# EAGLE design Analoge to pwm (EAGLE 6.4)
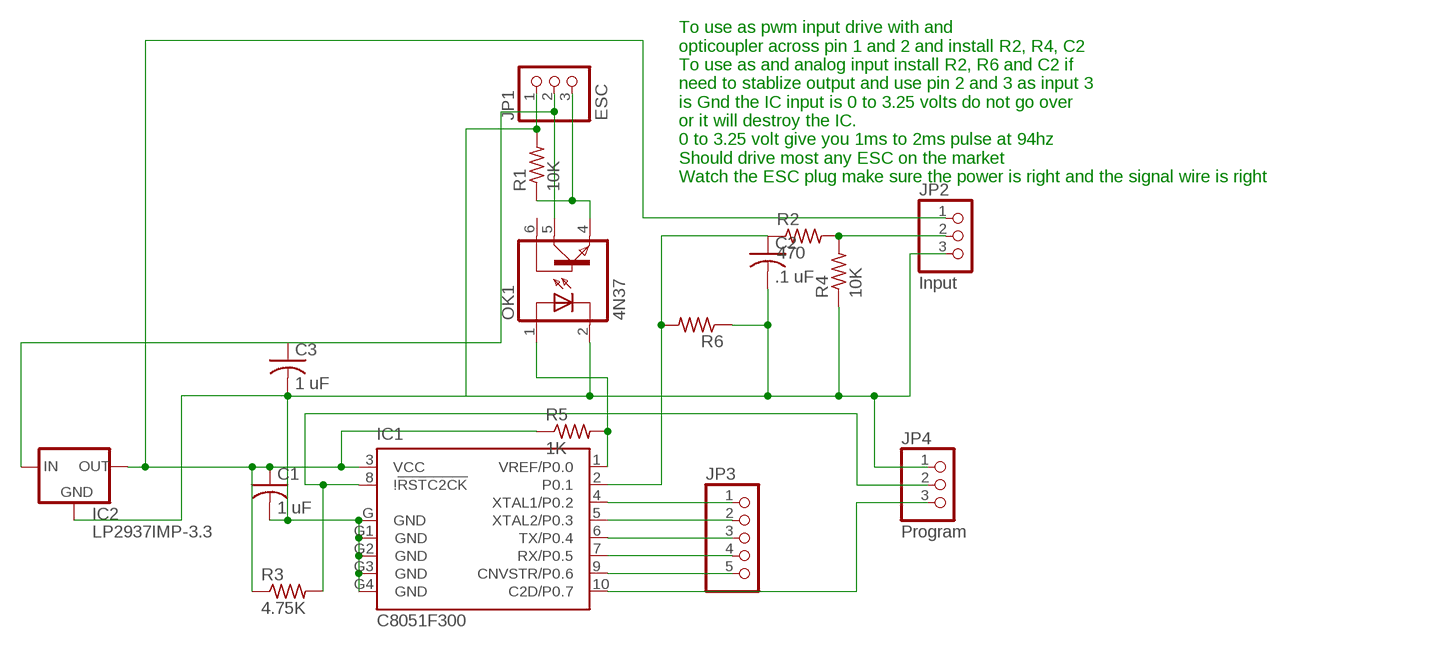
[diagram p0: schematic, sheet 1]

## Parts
C1  1 uF  C-USC0805  [C0805]
C2  .1 uF  C-USC0805  [C0805]
C3  1 uF  C-USC0805  [C0805]
IC1  C8051F300  [MLP11]
IC2  LP2937IMP-3.3  LP2950CDT-3.3  [DPACK]
JP1  ESC  PINHD-1X3  [1X03]
JP2  Input  PINHD-1X3  [1X03]
JP3  PINHD-1X5  [1X05]
JP4  Program  PINHD-1X3  [1X03]
OK1  4N37  [DIL06]
R1  10K  R-US_R0805  [R0805]
R2  470  R-US_R0805  [R0805]
R3  4.75K  R-US_M0805  [M0805]
R4  10K  R-US_R0805  [R0805]
R5  1K  R-US_R0805  [R0805]
R6  R-US_R0805  [R0805]

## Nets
N$1: IC1.10(C2D/P0.7) JP4.3
N$2: IC1.8(!!RSTC2CK) JP4.2 R3.2
N$4: IC1.1(VREF/P0.0) OK1.1(A) R5.2
N$6: C3.1 IC2.1(IN) JP1.2 OK1.5(COL)
N$7: JP1.3 OK1.4(EMI) R1.1
N$8: C1.2 C2.2 C3.2 IC1.G1(GND) IC1.G2(GND) IC1.G3(GND) IC1.G4(GND) IC1.G(GND) IC2.4(GND) JP1.1 JP2.3 JP4.1 OK1.2(C) R1.2 R4.1 R6.1
N$9: C2.1 IC1.2(P0.1) R2.1 R6.2
N$10: JP2.2 R2.2 R4.2
N$12: IC1.4(XTAL1/P0.2) JP3.1
N$13: IC1.5(XTAL2/P0.3) JP3.2
N$14: IC1.6(TX/P0.4) JP3.3
N$15: IC1.7(RX/P0.5) JP3.4
N$16: IC1.9(CNVSTR/P0.6) JP3.5
N$17: C1.1 IC1.3(VCC) IC2.3(OUT) JP2.1 R3.1 R5.1
Unconnected: OK1.6(BAS)

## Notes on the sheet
- To use as pwm input drive with and 
  opticoupler across pin 1 and 2 and install R2, R4, C2  
  To use as and analog input install R2, R6 and C2 if
  need to stablize output and use pin 2 and 3 as input 3 
  is Gnd the IC input is 0 to 3.25 volts do not go over
  or it will destroy the IC.
  0 to 3.25 volt give you 1ms to 2ms pulse at 94hz
  Should drive most any ESC on the market
  Watch the ESC plug make sure the power is right and the signal wire is right

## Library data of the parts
C1-C3 = resistor:C-US: CAPACITOR, American symbol
IC1 = silabs:C8051F30*: 25 MIPS, 8 kB Flash, 8-Bit ADC, 11-Pin Mixed-Signal MCU Source: http://www.silabs.com/products/microcontroller .. C8051F30xrev2_3.pdf; MPN: C8051F300-GM; OC_FARNELL: 4128310; OC_NEWARK: 96K8386
IC2 = v-reg:LP2950?*: Source: http://cache.national.com/ds/LP/LP2950.pdf
JP1 JP2 JP4 = pinhead:PINHD-1X3: PIN HEADER
JP3 = pinhead:PINHD-1X5: PIN HEADER
OK1 = optocoupler:4N37: OPTO COUPLER Source: http://www.fairchildsemi.com/pf/4N/4N35-M.html; MF: FAIRCHILD SEMICONDUCTOR; MPN: 4N37; OC_FARNELL: 1612456; OC_NEWARK: 72K9948
R1-R6 = resistor:R-US_: RESISTOR, American symbol

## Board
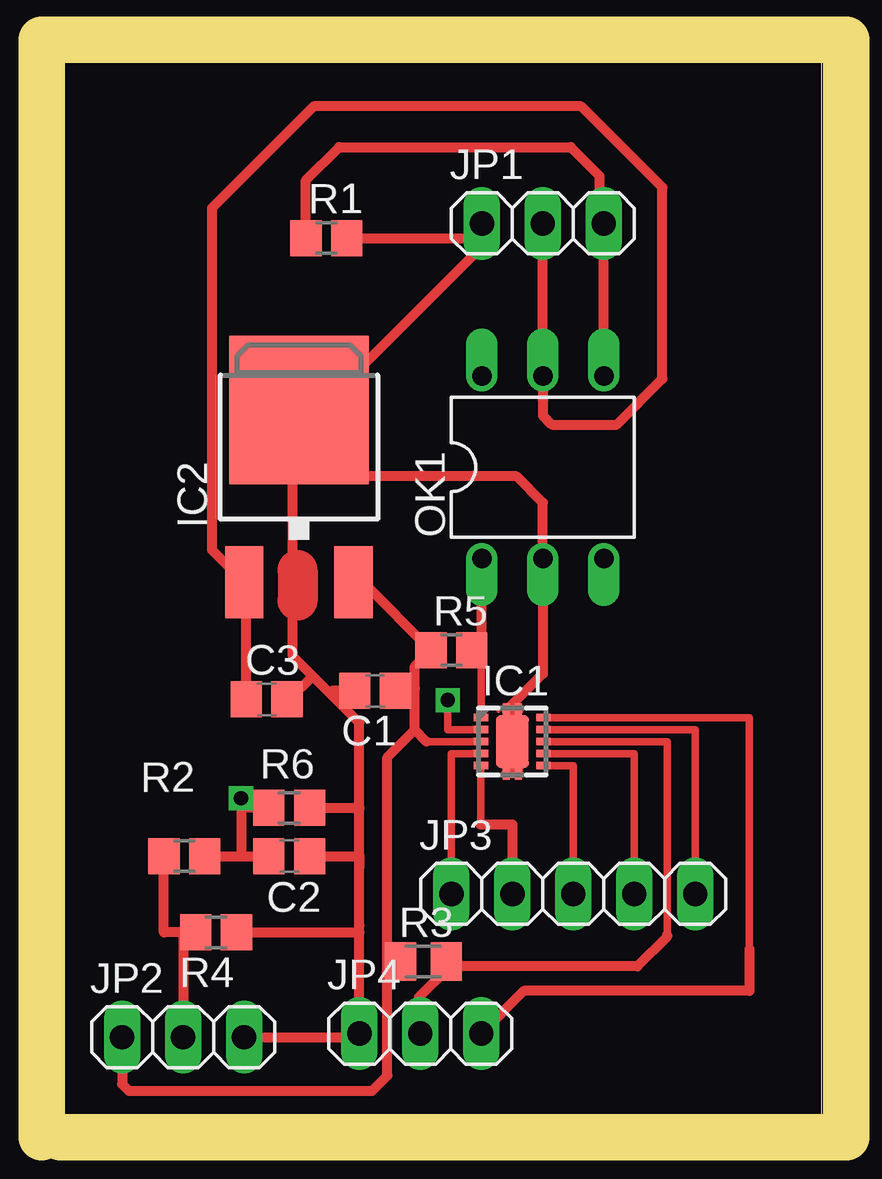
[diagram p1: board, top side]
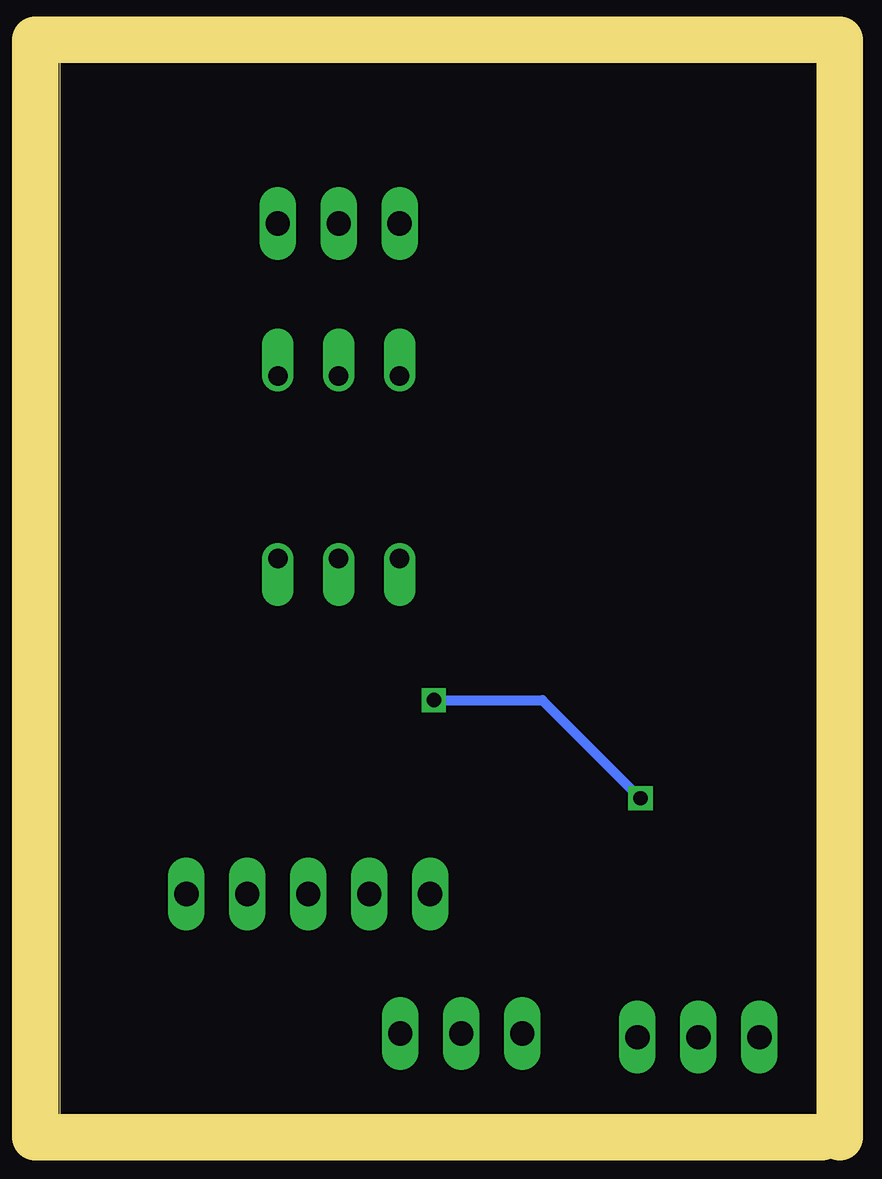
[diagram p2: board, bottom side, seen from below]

Size 31.73 x 44.12 mm. Coordinates in mm from the lower left corner, seen from the top.
Outline: 0,0 31.73,0 31.73,44.12 0,44.12 0,0
Copper layers (1*16): Top 0.035mm / dielectric 1.5mm / Bottom 0.035mm
Design rules "default": minimum track width 10mil, minimum drill 24mil, track to track 8mil, track to pad 8mil, pad to pad 8mil, via to via 8mil, smd to smd 8mil, copper to edge 40mil, drill to drill 8mil, minimum pad ring 10mil, minimum via ring 8mil, stop-mask expansion 4mil, vias tented up to drill 0mil, thermal gap 10mil
Milling: 4 lines

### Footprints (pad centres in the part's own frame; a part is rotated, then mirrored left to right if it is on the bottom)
C0805 = smd 1.3 x 1.5: 1 -0.85,0; 2 0.85,0
MLP11 = smd 0.6 x 0.3: 1 -1.3,1; 2 -1.3,0.5; 3 -1.3,0; 4 -1.3,-0.5; 5 -1.3,-1; 6 1.3,-1; 7 1.3,-0.5; 8 1.3,0; 9 1.3,0.5; 10 1.3,1 | smd 1.36 x 2.2: G 0,0 | smd 0.3 x 0.6: G1 -0.25,1.3; G2 0.25,1.3; G3 -0.25,-1.3; G4 0.25,-1.3
DPACK = smd 1.6 x 3: 1 -2.28,-4.8; 3 2.28,-4.8 | smd 5.8 x 6.2: 4 0,2.38
1X03 = drill 1.016 long: 1 -2.54,0; 2 0,0; 3 2.54,0
1X05 = drill 1.016 long: 1 -5.08,0; 2 -2.54,0; 3 0,0; 4 2.54,0; 5 5.08,0
DIL06 = drill 0.813 offset: 1 -2.54,-3.81; 2 0,-3.81; 3 2.54,-3.81; 4 2.54,3.81; 5 0,3.81; 6 -2.54,3.81
R0805 = smd 1.3 x 1.5: 1 -0.85,0; 2 0.85,0
M0805 = smd 1.3 x 1.6: 1 -0.95,0; 2 0.95,0

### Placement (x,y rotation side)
C1  13.13,17.83 180 top
C2  9.55,10.95 0 top
C3  8.61,17.48 0 top
IC1  18.85,15.72 0 top
IC2  9.96,27.15 0 top
JP1  20.12,37.31 0 top
JP2  5.13,3.4 0 top
JP3  21.39,9.37 0 top
JP4  15.01,3.56 0 top
OK1  20.12,27.15 0 top
R1  11.1,36.7 0 top
R2  5.18,10.95 180 top
R3  15.14,6.55 0 top
R4  6.5,7.77 180 top
R5  16.31,19.53 0 top
R6  9.55,12.95 180 top

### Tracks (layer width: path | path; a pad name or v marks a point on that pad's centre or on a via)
N$1
  Top 0.305: IC1.10 28.73,16.72 28.73,7.09
  Top 0.406: 28.73,7.09 28.73,5.33 19.33,5.33 JP4.3
N$2
  Top 0.305: IC1.8 25.3,15.72 25.3,7.67
  Top 0.406: 25.3,7.67 25.3,7.59 24.05,6.35 16.23,6.35 16.17,6.29 | 16.17,6.29 14.96,5.08 14.96,3.61 JP4.2 | R3.2 16.17,6.55 16.17,6.29
N$3
  Top 1.676: 9.91,22.86 9.91,21.59
N$4
  Top 0.305: 17.55,19.53 IC1.1
  Top 0.406: OK1.1 17.55,23.34 17.55,19.53 R5.2
N$6
  Top 0.406: JP1.2 OK1.5 20.12,29.31 20.5,28.93 23.19,28.93 25.09,30.84 25.09,38.81 21.72,42.19 10.57,42.19 6.33,37.95 6.33,23.7 IC2.1 7.76,22.27 C3.1
N$7
  Top 0.406: OK1.4 JP1.3 22.48,37.49 22.48,39.29 21.29,40.49 11.63,40.49 10.25,39.1 R1.1
N$8
  Top 0.406: IC1.G3 IC1.G4 19.1,15.47 IC1.G 18.85,16.77 IC1.G2 IC1.G1 20.12,18.54 OK1.2 20.12,25.68 19.02,26.77 12.72,26.77 10.36,29.13 | 10.36,29.13 IC2.4 | 12.47,8.05 JP4.1 12.32,3.4 JP2.3 | 12.47,8.05 12.47,10.49 | 12.47,10.49 12.47,12.93 | 12.47,12.93 12.47,16.51 11.24,17.74 | 11.24,17.74 10.53,18.45 | 10.53,18.45 9.7,19.28 9.7,28.47 9.99,28.77 | 9.99,28.77 10.36,29.13 | 9.99,28.77 17.58,36.35 JP1.1 16.97,36.7 R1.2 | C3.2 9.55,17.48 10.53,18.45 | C1.2 11.33,17.83 11.24,17.74 | R4.1 12.47,7.77 12.47,8.05 | C2.2 12.47,10.95 12.47,10.49 | R6.1 12.47,12.95 12.47,12.93
N$9  (via drill 0.6)
  Top 0.305: IC1.2 16.15,16.22 v16.15,17.45
  Top 0.406: R2.1 7.59,10.95 | 7.59,10.95 C2.1 | 7.59,10.95 7.54,11 v7.54,13.36 7.54,12.95 R6.2
  Bottom 0.406: v16.15,17.45 11.63,17.45 v7.54,13.36
N$10
  Top 0.406: JP2.2 5.13,7.77 R4.2 4.33,7.77 R2.2
N$12
  Top 0.305: IC1.4 16.31,15.22 JP3.1
N$13
  Top 0.254: IC1.5 17.53,14.72
  Top 0.305: 17.53,14.72 17.53,12.27
  Top 0.406: 17.53,12.27 18.85,12.27 JP3.2
N$14
  Top 0.305: IC1.6 21.39,14.72 JP3.3
N$15
  Top 0.305: IC1.7 23.93,15.22 JP3.4
N$16
  Top 0.305: IC1.9 26.47,16.22 JP3.5
N$17
  Top 0.305: IC1.3 15.27,15.72
  Top 0.406: IC2.3 12.64,22.35 R5.1 14.78,18.86 14.78,17.93 | 15.27,15.72 14.78,16.2 | 14.78,16.2 14.78,17.93 | C1.1 14.68,17.83 14.78,17.93 | JP2.1 2.59,1.45 2.87,1.17 13.01,1.17 13.64,1.8 13.64,6.45 | 13.64,6.45 13.64,15.06 14.78,16.2 | R3.1 13.64,6.55 13.64,6.45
